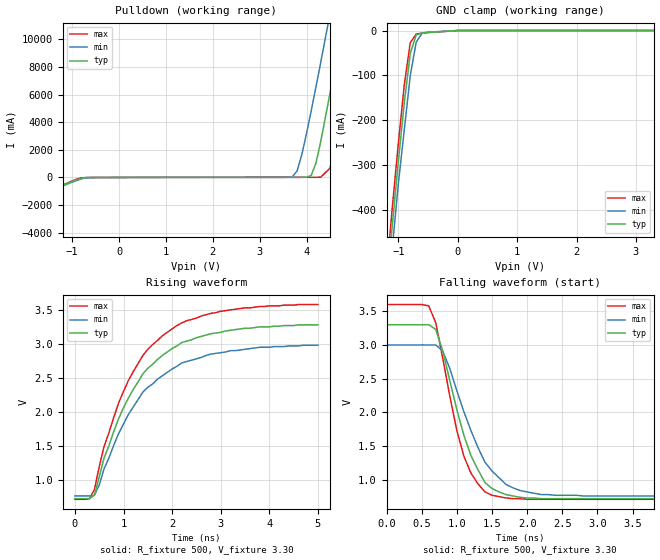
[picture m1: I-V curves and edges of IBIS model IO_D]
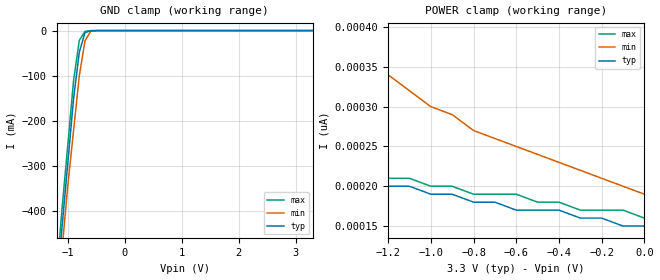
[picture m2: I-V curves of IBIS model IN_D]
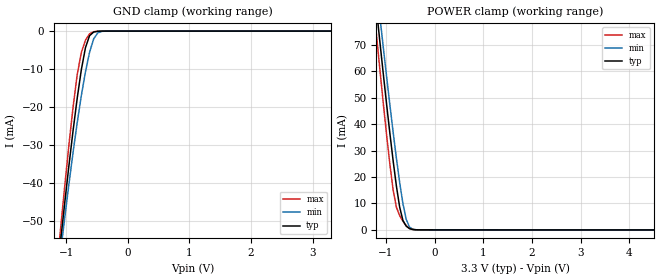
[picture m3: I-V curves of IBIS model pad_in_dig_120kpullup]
| Integrated Devices Technolgy, Inc
[Ibis Ver]   4.0
[File Name]   9qxl2000b.ibs
[File Rev]  1.2
|[Date]   April 22, 2018
|[Date]   May 15, 2019
[Date]   July 10, 2019
[Source] Integrated Device Technology, Inc.
[Notes]   Rev 1.2 created by LFP
[Disclaimer] Integrated Device Technology, Inc. ("IDT") hereby grants the
   user of this IBIS model a non-exclusive, nontransferable
   license to use this IBIS model under the following terms. The
   user is granted this license only to use the IBIS model and is
   not granted rights to sell, copy (except as needed to run the
   IBIS model), rent, lease or sub-license the IBIS model in
   whole or in part, or in modified form to anyone. The User may
   modify the IBIS model to suit its specific applications, but
   rights to derivative works and such modifications shall belong
   to IDT. This IBIS model is provided on an AS IS" basis and IDT
   makes absolutely no warranty with respect to the information
   contained herein. IDT DISCLAIMS AND CUSTOMER WAIVES ALL
   WARRANTIES, EXPRESS AND IMPLIED, INCLUDING WARRANTIES OF
   MERCHANTABILITY AND FITNESS FOR A PARTICULAR PURPOSE. THE
   ENTIRE RISK AS TO QUALITY AND PERFORMANCE IS WITH THE USER
   ACCORDINGLY, IN NO EVENT SHALL IDT BE LIABLE FOR ANY DIRECT OR
   INDIRECT DAMAGES, WHETHER IN CONTRACT OR TORT, INCLUDING ANY
   LOST PROFITS OR OTHER INCIDENTAL, CONSEQUENTIAL, EXEMPLARY, OR
   PUNITIVE DAMAGES ARISING OUT OF THE USE OR APPLICATION OF THE
   IBIS model. Further, IDT reserves the right to make changes
   without notice to any product herein to improve reliability,
   function, or design. IDT does not convey any license under
   patent rights or any other intellectual property rights,
   including those of third parties. IDT is not obligated to
   provide maintenance or support for the licensed IBIS model.
[Disclaimer]   (C) Copyright Integrated Device Technology, Inc. 2010 All
   rights reserved
|   COMPONENT: 9qxl2000b
[Component]   9qxl200b
[Manufacturer]   Integrated Device Technology, Inc.
[Package]
| variable   typ   min   max
R_pkg   81.10m   62.20m   100.00m
L_pkg   6.70nH   4.90nH   8.50nH
C_pkg   0.53pF   0.21pF   0.85pF
[Pin]   signal_name   model_name   R_pin   L_pin   C_pin
1   VDDA   POWER
2   GNDA   GND
3   NC   NC
4   NC   NC
5   NC   NC
6   CK_POWERGD/PD#   pad_in_dig_120kpullup
7   GND   GND
8   VDD   POWER
9   DIF_IN   pad_vprog_033
10   DIF_IN#   pad_vprog_033
11   SMB_A0_tri   pad_in_snbk_pullmid
12   SMBDAT   IO_D
13   SMBCLK   IN_D
14   SMB_A1_tri   pad_in_snbk_pullmid
15   NC   NC
16   NC   NC
17   DIF_19#   OUT
18   DIF_19   OUT
19   DIF_0   OUT
20   DIF_0#   OUT
21   VDD   POWER
22   DIF_1   OUT
23   DIF_1#   OUT
24   DIF_2   OUT
25   DIF_2#   OUT
26   GND   GND
27   DIF_3   OUT
28   DIF_3#   OUT
29   DIF_4   OUT
30   DIF_4#   OUT
31   VDD   POWER
32   DIF_5   OUT
33   DIF_5#   OUT
34   OE5#   pad_in_dig
35   DIF_6   OUT
36   DIF_6#   OUT
37   OE6#   pad_in_dig
38   DIF_7   OUT
39   DIF_7#   OUT
40   OE7#   pad_in_dig
41   DIF_8   OUT
42   DIF_8#   OUT
43   OE8#   pad_in_dig
44   GND   GND
45   VDD   POWER
46   DIF_9   OUT
47   DIF_9#   OUT
48   OE9#   pad_in_dig
49   DIF_10   OUT
50   DIF_10#   OUT
51   OE10#   pad_in_dig
52   DIF_11   OUT
53   DIF_11#   OUT
54   OE_11#   pad_in_dig
55   DIF_12   OUT
56   DIF_12#   OUT
57   OE12#   pad_in_dig
58   VDD   POWER
59   DIF_13   OUT
60   DIF_13#   OUT
61   DIF_14   OUT
62   DIF_14#   OUT
63   GND   GND
64   DIF_15   OUT
65   DIF_15#   OUT
66   DIF_16   OUT
67   DIF_16#   OUT
68   VDD   POWER
69   DIF_17   OUT
70   DIF_17#   OUT
71   DIF_18   OUT
72   DIF_18#   OUT
[Diff Pin]   inv_pin   vdiff   tdelay_typ
9   10   NA   NA
18   17   NA   NA
19   20   NA   NA
22   23   NA   NA
24   25   NA   NA
27   28   NA   NA
29   30   NA   NA
32   33   NA   NA
35   36   NA   NA
38   39   NA   NA
41   42   NA   NA
46   47   NA   NA
49   50   NA   NA
52   53   NA   NA
55   56   NA   NA
59   60   NA   NA
61   62   NA   NA
64   65   NA   NA
66   67   NA   NA
69   70   NA   NA
71   72   NA   NA
[Model Selector] OUT
pad_lpo_dbq_85   Nominal 42.5 ohm output impedance
pad_lpo_dbq_85m5  Nominal 42.5 ohm output impedance minus 5%
pad_lpo_dbq_85p5  Nominal 42.5 ohm output impedance plus 5%
| Models and submodels in the file (9): IO_D (I/O_open_drain), IN_D (Input), pad_in_dig_120kpullup (Input), pad_vprog_033 (Input), pad_in_snbk_pullmid (Input), pad_lpo_dbq_85 (Output), pad_lpo_dbq_85m5 (Output), pad_lpo_dbq_85p5 (Output), pad_in_dig (Input)
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|   Model IO_D
[Model]   IO_D
Model_type   I/O_open_drain
Polarity   Non-Inverting
Enable   Active-High
Vinl =   .300V
Vinh =   2.00V
Vmeas =   0.350V
Cref =   2.00pF
Rref =   0.000
Vref =   0.350V
C_comp   3.40pF   2.85pF   3.95pF
[Temperature Range]   27.00   70.00   0.000
[Voltage Range]   3.30V   3.00V   3.60V
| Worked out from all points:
|   slope of the pulldown table from 0 to 0.495 V, typ, clamps not added: 131 ohm
|   GND clamp passes 1 mA (typ) near -0.12 V on its own axis
|   rising waveform, R_fixture 500, V_fixture 3.30: 20-80 % time 1.13ns typ, 1.18ns min, 1.1ns max; typ from 0.72 V to 3.28 V
|   falling waveform, R_fixture 500, V_fixture 3.30: 20-80 % time 430ps typ, 510ps min, 367ps max; typ from 3.3 V to 0.72 V
[Pulldown]
| voltage   I(typ)   I(min)   I(max)
-3.3V     -3.78A     -3.65A     -3.87A
-800mV    -50.99mA   -100mA     -26.91mA
3.7V      9.44mA     53.55mA    11.23mA
3.8V      10.07mA    490mA      11.25mA
3.9V      12.32mA    1.67A      11.27mA
4.1V      150mA      4.83A      11.65mA
4.3V      2.56A      8.29A      17.33mA
4.5V      6.09A      11.85A     670mA
4.7V      9.81A      15.47A     3.91A
4.9V      13.62A     19.11A     7.69A
5.1V      17.46A     22.78A     11.6A
6.6V      46.76A     50.55A     41.81A
[GND_clamp]
| voltage   I(typ)   I(min)   I(max)
-3.3V     -3.78A     -3.65A     -3.87A
-1.2V     -570mA     -610mA     -540mA
-1.1V     -430mA     -480mA     -390mA
-1V       -290mA     -340mA     -250mA
-900mV    -160mA     -220mA     -120mA
-800mV    -50.99mA   -100mA     -26.91mA
-700mV    -9.68mA    -25.77mA   -7.84mA
-600mV    -5.33mA    -5.93mA    -5.63mA
0V        0A         0A         0A
3.3V      150pA      220pA      150pA
[Ramp]
| variable   typ   min   max
dV/dt_r   1.54/1.11n   1.33/1.16n   1.72/1.07n
dV/dt_f   1.55/0.42n   1.34/0.53n   1.73/0.36n
R_load = 500
[Rising Waveform]
R_fixture = 500
V_fixture = 3.30
V_fixture_min = 3.00
V_fixture_max = 3.60
| time   V(typ)   V(min)   V(max)
0s        720mV      760mV      710mV
300ps     720mV      760mV      720mV
400ps     770mV      770mV      850mV
600ps     1.32V      1.16V      1.49V
1ns       2.06V      1.82V      2.3V
1.4ns     2.56V      2.29V      2.83V
1.8ns     2.83V      2.53V      3.12V
2.2ns     3.02V      2.72V      3.31V
3ns       3.17V      2.87V      3.48V
5ns       3.28V      2.98V      3.58V
[Falling Waveform]
R_fixture = 500
V_fixture = 3.30
V_fixture_min = 3.00
V_fixture_max = 3.60
| time   V(typ)   V(min)   V(max)
0s        3.3V       3V         3.6V
600ps     3.3V       3V         3.58V
700ps     3.23V      3V         3.33V
800ps     2.91V      2.91V      2.8V
1ns       2.04V      2.32V      1.73V
1.1ns     1.66V      2.01V      1.35V
1.4ns     960mV      1.26V      820mV
1.7ns     780mV      930mV      730mV
2.2ns     720mV      780mV      710mV
5ns       720mV      760mV      710mV
|   Model IN_D
[Model]   IN_D
Model_type   Input
Polarity   Inverting
Enable   Active-High
Vinl =   1.00V
Vinh =   2.00V
C_comp   3.40pF   2.85pF   3.95pF
[Temperature Range]   27.00   70.00   0.000
[Voltage Range]   3.30V   3.00V   3.60V
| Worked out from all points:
|   GND clamp passes 1 mA (typ) near -0.62 V on its own axis
[GND_clamp]
| voltage   I(typ)   I(min)   I(max)
-3.3V     -3.78A     -3.65A     -3.87A
-1.2V     -570mA     -610mA     -540mA
-1.1V     -430mA     -480mA     -390mA
-1V       -290mA     -340mA     -250mA
-900mV    -150mA     -220mA     -110mA
-800mV    -47.77mA   -100mA     -21.77mA
-700mV    -4.42mA    -22.5mA    -1.71mA
-600mV    -390uA     -1.83mA    -190uA
-500mV    -33.14uA   -140uA     -13.41uA
3.3V      150pA      220pA      150pA
[POWER_clamp]
| voltage   I(typ)   I(min)   I(max)
-3.3V     350pA      1.67nA     300pA
-2.6V     280pA      890pA      270pA
-2.5V     280pA      820pA      260pA
-2.3V     260pA      700pA      260pA
-2.2V     250pA      640pA      250pA
-1.5V     220pA      400pA      220pA
-1.4V     210pA      380pA      220pA
-1V       190pA      300pA      200pA
-800mV    180pA      270pA      190pA
-600mV    170pA      250pA      190pA
-400mV    170pA      230pA      180pA
0V        150pA      190pA      160pA
|   Model pad_in_dig_120kpullup
[Model] pad_in_dig_120kpullup
Model_type Input
Vinl =   1.00V
Vinh =   2.00V
Polarity   Non-Inverting
C_comp   2.086pF   1.985pF   2.159pF
C_comp_pullup   1.049pF   0.980pF   1.113pF
[Temperature Range]   65.000   0.125k   -10.000
[Voltage Range]   3.300V   3.135V   3.465V
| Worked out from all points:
|   GND clamp passes 1 mA (typ) near -0.61 V on its own axis
|   POWER clamp passes 1 mA (typ) near -0.56 V on its own axis
[GND_clamp]
|Voltage   I(typ)   I(min)   I(max)
-3.3V     -432.5mA   -402.6mA   -464.3mA
-1.089V   -55.06mA   -58mA      -51.84mA
-1.022V   -45.06mA   -48.99mA   -40.67mA
-888mV    -26.23mA   -31.96mA   -20.04mA
-821mV    -17.71mA   -24.15mA   -11.5mA
-754mV    -10.2mA    -17.01mA   -5.648mA
-687mV    -4.38mA    -10.73mA   -2.405mA
-620mV    -1.197mA   -5.575mA   -730.9uA
-553mV    -247.7uA   -2.026mA   -149.1uA
-486mV    -49.14uA   -452.7uA   -22.56uA
-352mV    -1.583uA   -12.19uA   -251.1nA
3.3V      0A         0A         0A
[POWER_clamp]
|Voltage   I(typ)   I(min)   I(max)
-3.3V     496.3mA    485.4mA    509mA
-1.256V   94.12mA    102.6mA    85.06mA
-1.189V   82.11mA    91.16mA    72.29mA
-1.122V   70.29mA    79.87mA    59.76mA
-1.055V   58.7mA     68.76mA    47.54mA
-854mV    26.05mA    36.89mA    15.05mA
-787mV    16.51mA    27.04mA    8.532mA
-720mV    8.56mA     17.88mA    5.374mA
-653mV    3.538mA    9.889mA    3.235mA
-586mV    1.409mA    3.998mA    1.586mA
-519mV    499.1uA    1.079mA    539.8uA
6.6V      -25.49uA   -17.43uA   -38.26uA
